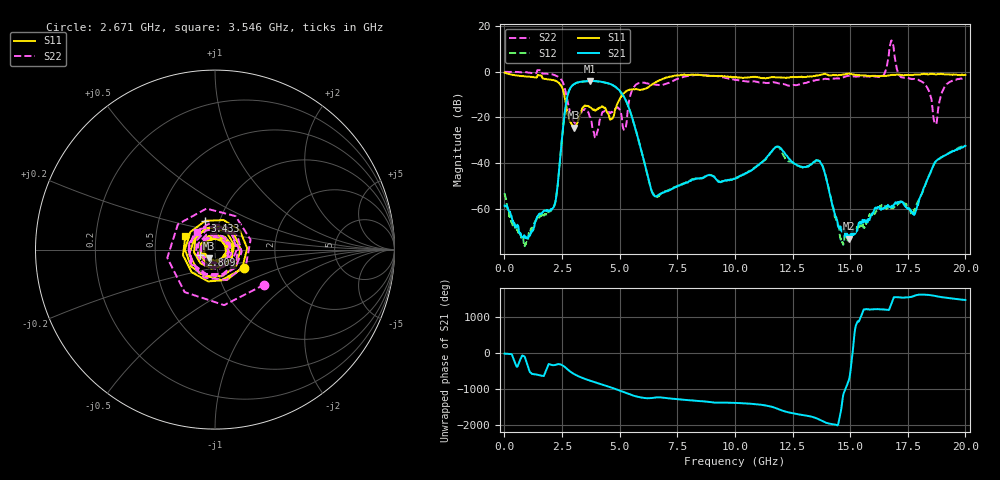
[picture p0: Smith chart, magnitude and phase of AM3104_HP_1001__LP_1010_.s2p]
!Created with skrf (http://scikit-rf.org).
# Hz S RI R 50.0
!freq ReS11 ImS11 ReS21 ImS21 ReS12 ImS12 ReS22 ImS22
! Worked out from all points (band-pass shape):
!   1601 points, 10 MHz to 20 GHz, reference 50 ohm
!   highest |S21| = -4.01 dB at 3.708 GHz (marker M1); lowest = -72.9 dB at 14.95 GHz (marker M2)
!   |S21| within 3 dB of the highest: 2.869 GHz to 4.868 GHz (1.999 GHz wide, 51.7 % of centre)
!   lowest |S11| = -24.5 dB at 3.021 GHz (marker M3), VSWR 1.13, Z = 46.4 - j4.51 ohm
!   |S11| at or under -10 dB: 2.595 GHz to 5.132 GHz (2.537 GHz wide, 65.7 % of centre)
!   |S22| runs from -29.0 to 13.6 dB; largest |S21 - S12| = 0.051
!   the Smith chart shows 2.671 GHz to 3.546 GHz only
!   S11 on the Smith chart (normalised r, x): 2.671 GHz: 1.36, -0.28; 2.809 GHz: 0.85, -0.06; 3.433 GHz: 0.85, +0.28; 3.546 GHz: 0.71, +0.11
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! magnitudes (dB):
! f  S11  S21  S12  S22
! 10 MHz  -0.4  -58.5  -53.0  0.0
! 922 MHz  -2.0  -72.4  -75.2  -0.2
! 2.084 GHz  -3.6  -59.8  -59.3  -1.2
! 2.671 GHz  -14.3  -14.1  -14.1  -9.4
! 2.809 GHz  -21.1  -8.2  -8.2  -16.1
! 3.021 GHz  -24.5  -5.5  -5.5  -22.0
! 3.346 GHz  -16.9  -4.4  -4.4  -17.6
! 3.433 GHz  -15.4  -4.2  -4.3  -16.7
! 3.546 GHz  -14.9  -4.1  -4.2  -16.9
! 3.708 GHz  -15.4  -4.0  -4.1  -19.7
! 5.17 GHz  -9.6  -10.6  -10.6  -25.1
! 5.67 GHz  -7.7  -24.4  -24.4  -6.1
! 6.682 GHz  -4.0  -53.9  -54.5  -5.8
! 10.01 GHz  -2.5  -46.8  -46.9  -3.6
! 11.83 GHz  -2.5  -32.8  -32.8  -5.0
! 13.34 GHz  -2.1  -40.2  -40.2  -4.1
! 14.95 GHz  -0.8  -72.9  -73.4  -1.7
! 16.68 GHz  -1.6  -59.1  -59.4  7.2
! 17.79 GHz  -1.4  -62.4  -60.3  -3.1
! 18.69 GHz  -1.1  -39.5  -39.6  -22.6
! 19.13 GHz  -1.2  -36.6  -36.5  -6.4
! 20 GHz  -1.4  -32.4  -32.0  -2.6
